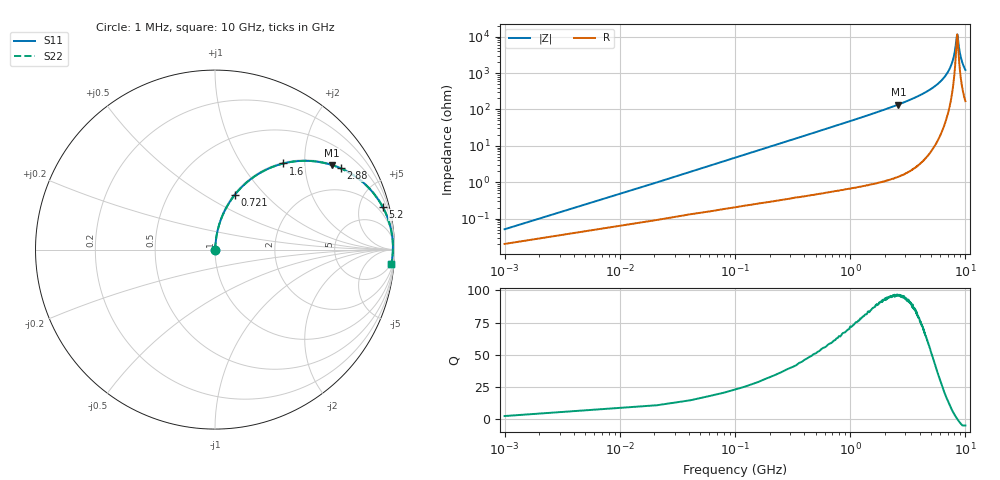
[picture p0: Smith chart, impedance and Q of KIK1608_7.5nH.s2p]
!version-2
!date-01.2022
!Series
# MHz S RI R 50
!Freq ReS11 ImS11 ReS21 ImS21 ReS12 ImS12 ReS22 ImS22
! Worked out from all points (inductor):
!   501 points, 1 MHz to 10 GHz, reference 50 ohm
!   read as one part in series: L = 7.5 nH near 41 MHz
!   highest Q = 96 at 2.62 GHz (marker M1), where L = 8.29 nH
!   self-resonance near 8.48 GHz
!   S11 on the Smith chart (normalised r, x): 1 MHz: 1.00, +0.00; 721 MHz: 1.01, +0.68; 1.6 GHz: 1.02, +1.56; 2.88 GHz: 1.03, +3.07; 5.2 GHz: 1.16, +7.83; 10 GHz: 4, -24
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1  0.000206 0.000471  0.9998 -0.000471  0.9998 -0.000471  0.000206 0.000471
61  0.00243 0.0286  0.9976 -0.0286  0.9976 -0.0286  0.00243 0.0286
101  0.00431 0.0473  0.9957 -0.0473  0.9957 -0.0473  0.00431 0.0473
141  0.00681 0.0659  0.9932 -0.0659  0.9932 -0.0659  0.00681 0.0659
241  0.0158 0.1115  0.9842 -0.1115  0.9842 -0.1115  0.0158 0.1115
361  0.0318 0.1644  0.9682 -0.1644  0.9682 -0.1644  0.0318 0.1644
721  0.1088 0.3033  0.8912 -0.3033  0.8912 -0.3033  0.1088 0.3033
1600  0.381 0.4799  0.619 -0.4799  0.619 -0.4799  0.381 0.4799
1680  0.4057 0.4854  0.5943 -0.4854  0.5943 -0.4854  0.4057 0.4854
2620  0.6493 0.472  0.3507 -0.472  0.3507 -0.472  0.6493 0.472
2880  0.6999 0.4531  0.3001 -0.4531  0.3001 -0.4531  0.6999 0.4531
3340  0.7737 0.4129  0.2263 -0.4129  0.2263 -0.4129  0.7737 0.4129
5020  0.9255 0.2532  0.0745 -0.2532  0.0745 -0.2532  0.9255 0.2532
5200  0.9345 0.2372  0.0655 -0.2372  0.0655 -0.2372  0.9345 0.2372
6680  0.9794 0.118  0.0205 -0.118  0.0205 -0.118  0.9794 0.118
7740  0.9903 0.0459  0.0097 -0.0459  0.0097 -0.0459  0.9903 0.0459
8080  0.9913 0.0248  0.00866 -0.0248  0.00866 -0.0248  0.9913 0.0248
8340  0.9915 0.0092  0.00851 -0.0092  0.00851 -0.0092  0.9915 0.0092
8520  0.9913 -0.00128  0.0087 0.00128  0.0087 0.00128  0.9913 -0.00128
8840  0.9904 -0.0193  0.00958 0.0193  0.00958 0.0193  0.9904 -0.0193
9100  0.9892 -0.0335  0.0108 0.0335  0.0108 0.0335  0.9892 -0.0335
10000  0.9824 -0.0791  0.0176 0.0791  0.0176 0.0791  0.9824 -0.0791
